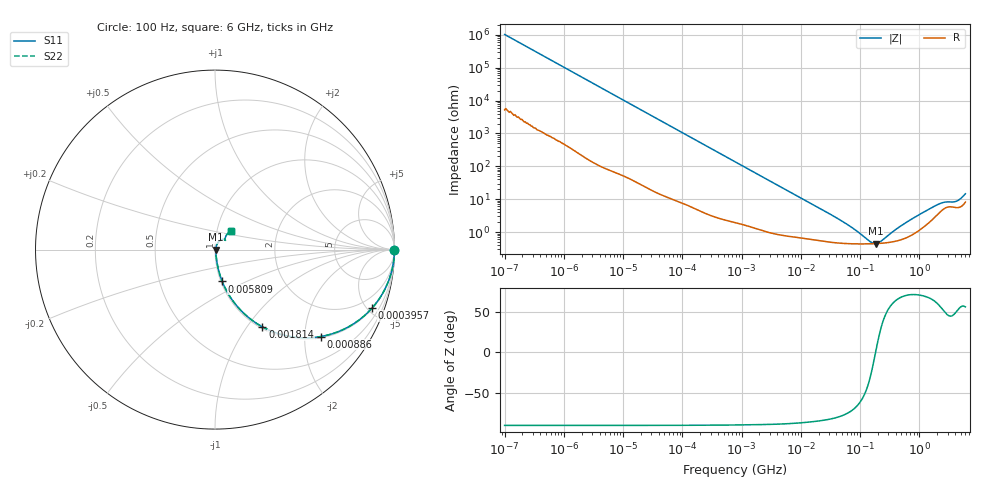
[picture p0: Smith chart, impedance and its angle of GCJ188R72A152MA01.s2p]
!Murata Part Number: GCJ188R72A152MA01
!These Parameters are Measured in Series Mode Connection
!Data Generated on Mar 13, 2026
!  o--ll--o
!Port1  Port2
!  o------o
!Operation Temp=25[degC], DC Bias Voltage=0[V]
!Freq. Start=100[Hz] Stop=6[GHz] 401[Steps]
# Hz S RI R 50
!Freq.(Hz) S11(Real) S11(Imag) S21(Real) S21(Imag) S12(Real) S12(Imag) S22(Real) S22(Imag)
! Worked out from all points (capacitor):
!   401 points, 100 Hz to 6 GHz, reference 50 ohm
!   read as one part in series: C = 1.54 nF near 109 Hz
!   lowest |Z| = 444 mohm at 182.6 MHz (marker M1)
!   series resonance near 182.6 MHz, so ESL is about 490 pH
!   S11 on the Smith chart (normalised r, x): 100 Hz: open; 395.7 kHz: 1.05, -5.37; 886 kHz: 1.04, -2.41; 1.814 MHz: 1.02, -1.18; 5.809 MHz: 1.02, -0.37; 6 GHz: 1.16, +0.24
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100  1 -9.67e-05  5e-07 9.67e-05  5e-07 9.67e-05  1 -9.67e-05
2008  1 -0.00192  1.16e-05 0.00192  1.16e-05 0.00192  1 -0.00192
40335  0.9983 -0.0382  0.00168 0.0382  0.00168 0.0382  0.9983 -0.0382
141303  0.9815 -0.131  0.0185 0.131  0.0185 0.131  0.9815 -0.131
395726  0.8757 -0.325  0.1243 0.325  0.1243 0.325  0.8757 -0.325
774597  0.6524 -0.4692  0.3476 0.4692  0.3476 0.4692  0.6524 -0.4692
885955  0.5906 -0.4842  0.4094 0.4842  0.4094 0.4842  0.5906 -0.4842
1267578  0.4178 -0.4843  0.5822 0.4843  0.5822 0.4843  0.4178 -0.4843
1813585  0.2641 -0.4305  0.7359 0.4305  0.7359 0.4305  0.2641 -0.4305
3103719  0.1143 -0.305  0.8857 0.305  0.8857 0.305  0.1143 -0.305
5809218  0.0404 -0.1776  0.9596 0.1776  0.9596 0.1776  0.0404 -0.1776
1.555665e7  0.0107 -0.0692  0.9893 0.0692  0.9893 0.0692  0.0107 -0.0692
5.211241e7  0.00487 -0.0196  0.9951 0.0196  0.9951 0.0196  0.00487 -0.0196
1.459435e8  0.00436 -0.00277  0.9956 0.00277  0.9956 0.00277  0.00436 -0.00277
1.825626e8  0.00442 -3.5e-06  0.9956 3.5e-06  0.9956 3.5e-06  0.00442 -3.5e-06
2.183701e8  0.00451 0.0022  0.9955 -0.0022  0.9955 -0.0022  0.00451 0.0022
3.124326e8  0.00487 0.0069  0.9951 -0.0069  0.9951 -0.0069  0.00487 0.0069
6.395615e8  0.00733 0.0195  0.9927 -0.0195  0.9927 -0.0195  0.00733 0.0195
1.712697e9  0.0271 0.0498  0.9729 -0.0498  0.9729 -0.0498  0.0271 0.0498
2.562649e9  0.0507 0.0564  0.9493 -0.0564  0.9493 -0.0564  0.0507 0.0564
4.193612e9  0.0562 0.0589  0.9438 -0.0589  0.9438 -0.0589  0.0562 0.0589
6e9  0.0871 0.1025  0.9129 -0.1025  0.9129 -0.1025  0.0871 0.1025
